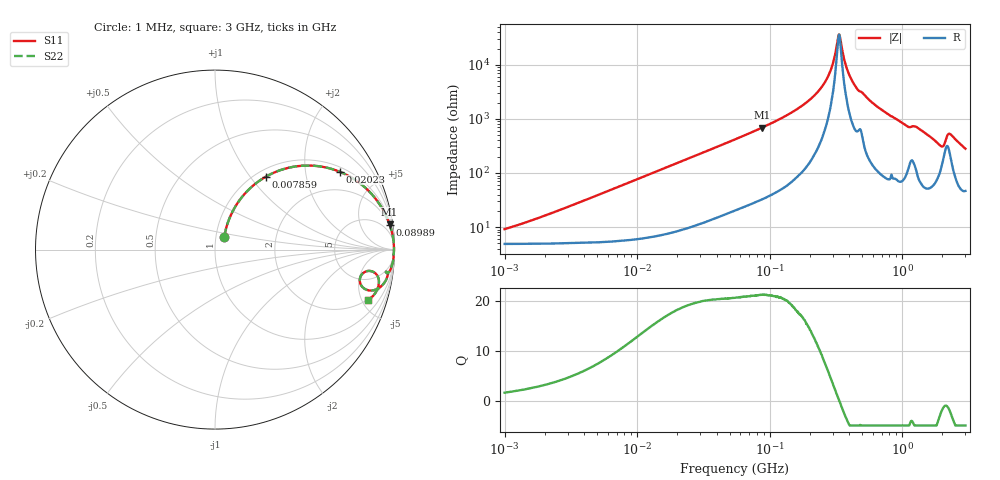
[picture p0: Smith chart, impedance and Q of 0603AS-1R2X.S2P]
!s-Parameter Generated by FASTRON Sdn. Bhd.
!FASTRON P/N : 0603AS-1R2X
!Keysight Technologies: E4991B_MY54100416_A.01.15
!Date created: Tue Oct 17 14:50:44 2023
!Version  : Rev01 Tue Oct 17 14:50:44 2023
!Data & Calibration Information:
!Freq	S11	S21	S12	S22
!PortZ  Port1:50+j0  Port2:50+j0
!When reading reference impedance value at option line is always used.
! Remarks : This data is being provided solely for informational purposes.
# Hz S dB R 50
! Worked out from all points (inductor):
!   1601 points, 1 MHz to 3 GHz, reference 50 ohm
!   read as one part in series: L = 1.23 uH near 1.917 MHz
!   highest Q = 21.2 at 87.23 MHz (marker M1), where L = 1.25 uH
!   self-resonance near 333.5 MHz
!   S11 on the Smith chart (normalised r, x): 1 MHz: 1.10, +0.16; 7.859 MHz: 1.11, +1.20; 20.23 MHz: 1.17, +3.08; 89.89 MHz: 2, +14; 3 GHz: 1.93, -5.56
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1000000  -21.18 53.6  -0.44 -4.2  -0.44 -4.2  -21.18 53.6
3804036  -11.31 64.6  -0.76 -15.5  -0.76 -15.5  -11.31 64.6
7858845  -6.07 55.0  -1.69 -29.7  -1.69 -29.7  -6.07 55.0
1.447069e7  -2.86 40.5  -3.73 -45.9  -3.73 -45.9  -2.86 40.5
2.023456e7  -1.73 32.0  -5.50 -54.9  -5.50 -54.9  -1.73 32.0
5.477226e7  -0.34 13.3  -12.77 -73.9  -12.77 -73.9  -0.34 13.3
8.723049e7  -0.15 8.2  -16.89 -79.1  -16.89 -79.1  -0.15 8.2
8.98892e7  -0.14 7.9  -17.18 -79.4  -17.18 -79.4  -0.14 7.9
1.475212e8  -0.06 4.3  -22.53 -82.7  -22.53 -82.7  -0.06 4.3
2.083556e8  -0.03 2.3  -27.83 -83.4  -27.83 -83.4  -0.03 2.3
2.771263e8  -0.02 0.9  -35.96 -79.3  -35.96 -79.3  -0.02 0.9
3.002264e8  -0.02 0.5  -40.55 -72.7  -40.55 -72.7  -0.02 0.5
3.268837e8  -0.02 0.1  -49.62 -34.9  -49.62 -34.9  -0.02 0.1
3.351655e8  -0.02 -0.0  -51.22 3.6  -51.22 3.6  -0.02 -0.0
3.836505e8  -0.03 -0.7  -38.44 75.0  -38.44 75.0  -0.03 -0.7
4.435663e8  -0.04 -1.4  -32.11 79.7  -32.11 79.7  -0.04 -1.4
7.925923e8  -0.08 -4.7  -21.64 81.6  -21.64 81.6  -0.08 -4.7
1.519029e9  -0.30 -10.4  -14.81 74.0  -14.81 74.0  -0.30 -10.4
1.931433e9  -1.12 -14.9  -11.33 56.3  -11.33 56.3  -1.12 -14.9
2.071593e9  -1.69 -11.0  -12.14 39.3  -12.14 39.3  -1.69 -11.0
2.289646e9  -0.78 -9.0  -15.26 55.7  -15.26 55.7  -0.78 -9.0
3e9  -0.95 -18.3  -9.95 62.2  -9.95 62.2  -0.95 -18.3
